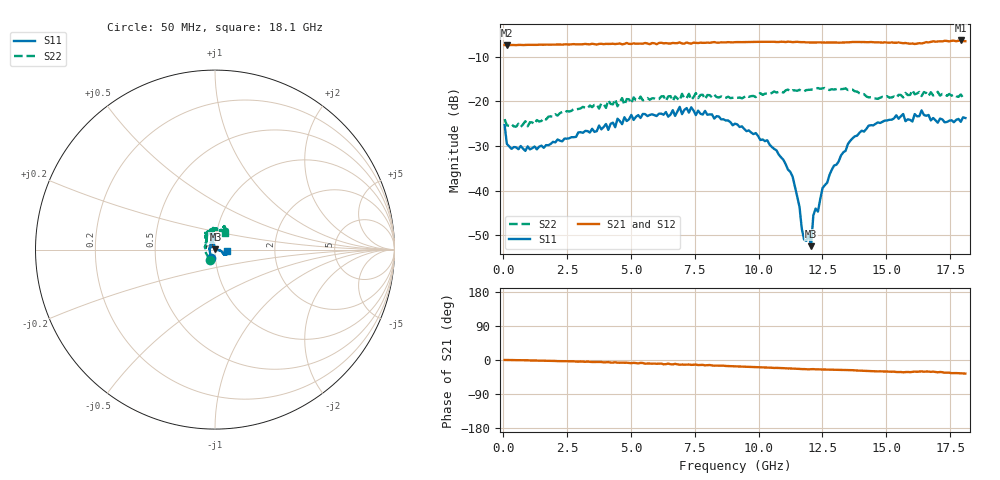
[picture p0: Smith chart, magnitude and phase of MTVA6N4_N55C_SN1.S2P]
! Network Analyzer HP8720D.06.14 Serial No. US36140669
!  6 Jul 2005  07:16:15
! Frequency  S11  S21  S12  S22
# HZ  S  DB R 50
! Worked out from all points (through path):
!   201 points, 50 MHz to 18.1 GHz, reference 50 ohm
!   highest |S21| = -6.40 dB at 17.92 GHz (marker M1); lowest = -7.5 dB at 140.2 MHz (marker M2)
!   group delay of S21, straight-line fit = 5.78 ps
!   lowest |S11| = -52.4 dB at 12.05 GHz (marker M3), VSWR 1.00, Z = 50.2 + j0.108 ohm
!   |S11| at or under -10 dB: start of sweep to end of sweep
!   |S22| runs from -25.7 to -17.0 dB; largest |S21 - S12| = 0.014
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5e7  -25.32 -116.0  -7.42 0.0  -7.45 0.0  -24.00 -118.0
1.4025e8  -29.54 -144.0  -7.46 0.0  -7.44 -0.1  -25.39 -158.9
1.3135e9  -30.75 153.1  -7.38 -1.5  -7.36 -1.5  -24.19 147.5
3.1185e9  -27.05 120.0  -7.24 -4.3  -7.28 -4.6  -21.25 128.2
6.09675e9  -22.78 98.3  -6.96 -9.8  -6.88 -10.0  -19.50 105.3
7.36025e9  -21.35 89.5  -7.10 -12.8  -6.97 -12.1  -19.68 98.6
9.075e9  -25.00 105.9  -6.78 -16.5  -6.75 -16.5  -19.18 78.5
1.097025e10  -33.08 102.4  -6.69 -21.6  -6.71 -21.8  -18.06 63.7
1.133125e10  -36.82 90.9  -6.77 -22.5  -6.74 -22.8  -17.53 64.0
1.17825e10  -50.92 20.1  -6.77 -24.0  -6.78 -24.4  -17.74 66.3
1.1963e10  -49.82 99.2  -6.84 -24.7  -6.88 -24.6  -17.44 69.6
1.205325e10  -52.39 26.6  -6.86 -24.2  -6.87 -24.5  -17.40 68.8
1.21435e10  -45.49 17.9  -6.86 -24.1  -6.80 -24.4  -17.34 68.8
1.2324e10  -44.67 6.4  -6.83 -24.7  -6.83 -25.0  -17.03 69.0
1.25045e10  -39.39 -8.7  -6.84 -25.1  -6.86 -25.3  -17.10 67.3
1.35875e10  -28.84 -13.6  -6.79 -26.7  -6.77 -27.0  -17.38 67.3
1.512175e10  -24.13 -26.8  -6.90 -30.8  -6.76 -30.9  -19.17 64.9
1.602425e10  -24.51 -10.2  -7.07 -31.2  -7.22 -32.6  -17.50 58.6
1.638525e10  -22.03 -5.9  -7.07 -30.1  -6.92 -30.0  -18.83 58.1
1.7017e10  -24.78 -2.9  -6.61 -32.5  -6.62 -33.3  -17.88 61.5
1.79195e10  -24.58 -7.2  -6.40 -35.2  -6.38 -35.7  -18.47 64.7
1.81e10  -23.74 -6.1  -6.56 -35.8  -6.68 -36.1  -19.08 58.5
